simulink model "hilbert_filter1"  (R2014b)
settings: Solver=ode45  StartTime=0.0  StopTime=10.0  RelTol=1e-3
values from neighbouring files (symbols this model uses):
  delta = nord/2    (= 32)    [hilbert_filter_1.m]    (also in hilbert_filter_2.m; hilbert_filter_3.m; inv_sinc_1.m = 25; komplexe_huelle_1.m)
  hd = Hd.numerator    [fdesign_1.m]    (also in grp_komp_1.m = fdesign.lowpass('N,Fp,Ap,Ast',nord,fr,dp,ds); hilbert_filter_1.m = design(d, 'equiripple'); hilbert_filter_2.m = design(d, 'equiripple'); hilbert_filter_3.m = design(d, 'equiripple'))
  k = 1    [hilbert_filter_1.m]    (also in hilbert_filter_2.m; komplexe_huelle_1.m; lattice_11.m = tf2latc(a); sgolay_1.m = 3)
  Ts = 1/fs    (= 0.001)    [abtast_fir_1.m]    (also in abtast_fir_2.m; abtast_fir_3.m; abtast_fir_4.m; hilbert_filter_1.m)

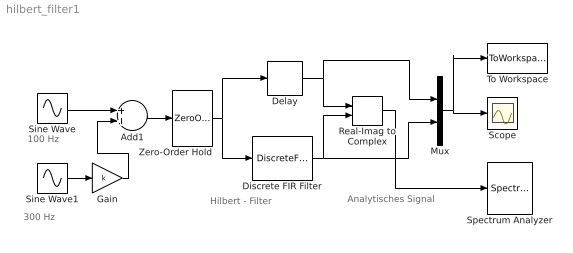
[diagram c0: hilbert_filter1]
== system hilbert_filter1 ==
  note: 300 Hz
  note: 100 Hz
  note: Hilbert - Filter
  note: Analytisches Signal
  Add1 : Sum
  Delay : Delay  DelayLength=delta  UseCircularBuffer=on  SampleTime=Ts
  Discrete FIR Filter : DiscreteFir  Coefficients=hd.numerator
  Gain : Gain  Gain=k
  Mux : Mux  Inputs=2
  Real-Imag to Complex : RealImagToComplex
  Scope : Scope
  Sine Wave : Sin  Frequency=2*pi*100  SampleTime=0
  Sine Wave1 : Sin  Frequency=2*pi*300  SampleTime=0
  Spectrum Analyzer : SpectrumAnalyzer
  To Workspace : ToWorkspace  VariableName=y  SaveFormat=Timeseries  SampleTime=-1
  Zero-Order Hold : ZeroOrderHold  SampleTime=Ts
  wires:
  Add1/1 -> Zero-Order Hold/1
  Sine Wave/1 -> Add1/1
  Sine Wave1/1 -> Gain/1
  Mux/1 -> To Workspace/1, Scope/1
  Discrete FIR Filter/1 -> Mux/2, Real-Imag to Complex/2
  Real-Imag to Complex/1 -> Spectrum Analyzer/1
  Zero-Order Hold/1 -> Discrete FIR Filter/1, Delay/1
  Delay/1 -> Mux/1, Real-Imag to Complex/1
  Gain/1 -> Add1/2
